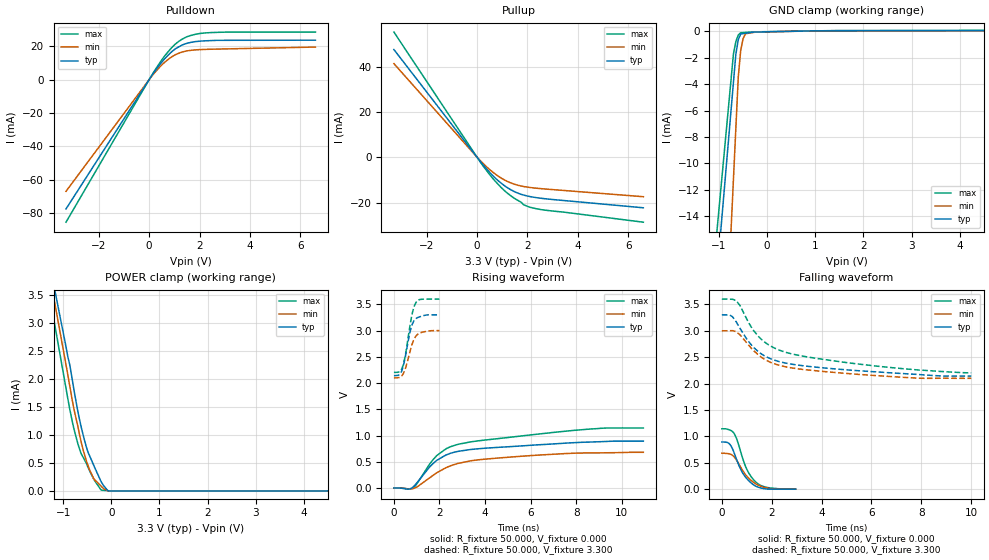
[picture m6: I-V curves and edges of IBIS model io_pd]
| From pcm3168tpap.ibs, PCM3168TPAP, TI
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[Model]   io_pd
Model_type I/O
Vinl=8.000E-01
Vinh=2.000E+00
Vref=0.000E+00
Rref=1.000E+06
Cref=0.000E+00
Vmeas=1.650E+00
C_comp   777.000fF   777.000fF   777.000fF
[Voltage Range]   3.300E+00   3.000E+00   3.600E+00
[POWER Clamp Reference]   3.300E+00   3.000E+00   3.600E+00
[GND Clamp Reference]   0.000E+00   0.000E+00   0.000E+00
[Pullup Reference]   3.300E+00   3.000E+00   3.600E+00
[Pulldown Reference]   0.000E+00   0.000E+00   0.000E+00
[Temperature Range]   25   105   -40
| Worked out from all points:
|   slope of the pulldown table from 0 to 0.495 V, typ, clamps not added: 47.9 ohm
|   slope of the pullup table from 0 to 0.495 V, typ, clamps not added: 75 ohm
|   GND clamp passes 1 mA (typ) near -0.62 V on its own axis
|   POWER clamp passes 1 mA (typ) near -0.58 V on its own axis
|   rising waveform, R_fixture 50.000, V_fixture 0.000: 20-80 % time 1.91ns typ, 2.48ns min, 2.8ns max; typ from 0.001 V to 0.893 V
|   falling waveform, R_fixture 50.000, V_fixture 0.000: 20-80 % time 570ps typ, 656ps min, 566ps max; typ from 0.893 V to 0.001 V
|   rising waveform, R_fixture 50.000, V_fixture 3.300: 20-80 % time 329ps typ, 362ps min, 321ps max; typ from 2.14 V to 3.3 V
|   falling waveform, R_fixture 50.000, V_fixture 3.300: 20-80 % time 2.02ns typ, 2.14ns min, 2.82ns max; typ from 3.3 V to 2.14 V
[GND Clamp]
-3.3V     -115.1mA   -212.3mA   -103.7mA
-700mV    -3.874mA   -11.24mA   -1.714mA
-650mV    -1.736mA   -7.37mA    -766.1uA
-600mV    -630.8uA   -3.503mA   -281.1uA
-550mV    -201uA     -1.481mA   -100.3uA
-500mV    -173.9uA   -551.7uA   -88.38uA
-450mV    -146.8uA   -176uA     -76.5uA
-225mV    -48.16uA   -44.71uA   -32uA
1V        44uA       32.79uA    39.81uA
6.6V      71.44uA    52.14uA    84.86uA
[Power Clamp]
-3.3V     12.83mA    13.4mA     13.34mA
-960mV    2.667mA    2.35mA     1.931mA
-900mV    2.393mA    2.064mA    1.638mA
-860mV    2.248mA    1.866mA    1.451mA
-760mV    1.731mA    1.402mA    1.057mA
-640mV    1.201mA    930.3uA    700.9uA
-580mV    984.6uA    720.8uA    594.8uA
-480mV    684.7uA    443.6uA    416.2uA
-360mV    448.8uA    211.8uA    202.8uA
-200mV    149.3uA    74.96uA    12.57uA
-60mV     0A         0A         0A
6.6V      0A         0A         0A
[Pullup]
-3.3V     47.49mA    41.29mA    55.2mA
180mV     -2.565mA   -2.087mA   -2.929mA
740mV     -9.368mA   -7.553mA   -10.81mA
1.06V     -12.33mA   -9.836mA   -14.46mA
1.3V      -14.1mA    -11.15mA   -16.68mA
1.74V     -16.33mA   -12.67mA   -19.79mA
1.84V     -16.66mA   -12.89mA   -20.9mA
2.34V     -17.8mA    -13.65mA   -22.68mA
6.6V      -22.3mA    -17.41mA   -28.65mA
[Pulldown]
-3.3V     -77.4mA    -66.86mA   -85.34mA
140mV     3.167mA    2.696mA    3.525mA
620mV     12.54mA    10.43mA    14.23mA
920mV     17.01mA    13.85mA    19.51mA
1.1V      18.97mA    15.3mA     22.02mA
1.5V      21.72mA    17.19mA    25.66mA
1.9V      22.83mA    17.86mA    27.34mA
2.2V      23.2mA     18.08mA    27.92mA
3.06V     23.53mA    18.38mA    28.44mA
6.6V      23.6mA     19.49mA    28.45mA
[Rising Waveform]
R_fixture = 50.000
V_fixture = 0.000
V_fixture_min = 0.000
V_fixture_max = 0.000
|  time   V(typ)   V(min)   V(max)
0s        731.5uV    760.4uV    415.8uV
600ps     -22.04mV   -15.56mV   -17.06mV
840ps     19.73mV    -11.36mV   2.595mV
1.56ns    396.4mV    191.2mV    451.3mV
1.89ns    529.4mV    292.7mV    620.4mV
2.33ns    636.8mV    395.6mV    756.8mV
2.86ns    702mV      473.6mV    837mV
3.98ns    757.7mV    549.5mV    913.1mV
7.91ns    864.3mV    663mV      1.099V
10.95ns   893.5mV    680.4mV    1.144V
[Falling Waveform]
R_fixture = 50.000
V_fixture = 0.000
V_fixture_min = 0.000
V_fixture_max = 0.000
|  time   V(typ)   V(min)   V(max)
0s        893.5mV    680.4mV    1.144V
280ps     869mV      671.5mV    1.127V
500ps     680.1mV    609mV      1.05V
610ps     540.2mV    535.8mV    934.3mV
810ps     327.1mV    374.7mV    621.8mV
980ps     212.2mV    259mV      399.3mV
1.18ns    117.5mV    163.6mV    234.7mV
1.39ns    51.16mV    94.02mV    125.1mV
1.83ns    2.195mV    20.3mV     31.75mV
2.96ns    731.5uV    760.4uV    415.8uV
[Rising Waveform]
R_fixture = 50.000
V_fixture = 3.300
V_fixture_min = 3.000
V_fixture_max = 3.600
|  time   V(typ)   V(min)   V(max)
0s        2.142V     2.099V     2.204V
250ps     2.164V     2.109V     2.22V
390ps     2.291V     2.164V     2.322V
520ps     2.545V     2.298V     2.576V
720ps     2.996V     2.623V     3.133V
790ps     3.102V     2.729V     3.298V
870ps     3.18V      2.823V     3.436V
970ps     3.23V      2.898V     3.537V
1.18ns    3.27V      2.96V      3.595V
2ns       3.3V       3V         3.6V
[Falling Waveform]
R_fixture = 50.000
V_fixture = 3.300
V_fixture_min = 3.000
V_fixture_max = 3.600
|  time   V(typ)   V(min)   V(max)
0s        3.3V       3V         3.6V
380ps     3.281V     3.002V     3.597V
580ps     3.167V     2.981V     3.568V
730ps     3.044V     2.923V     3.476V
1.02ns    2.828V     2.759V     3.202V
1.5ns     2.591V     2.529V     2.877V
1.95ns    2.471V     2.403V     2.712V
2.6ns     2.384V     2.313V     2.587V
6.22ns    2.221V     2.15V      2.33V
10.01ns   2.142V     2.099V     2.204V
[Ramp]
dV/dt_r   5.2957E-01/1.8780E-09   4.0232E-01/2.4679E-09   6.7583E-01/2.8000E-09
dV/dt_f   6.9475E-01/2.0178E-09   5.4036E-01/2.1344E-09   8.3763E-01/2.8124E-09
R_load = 50
